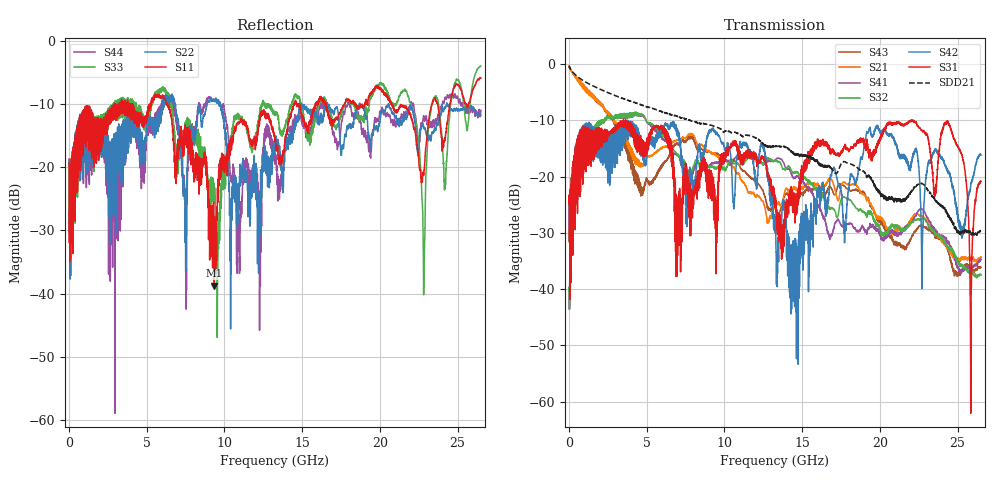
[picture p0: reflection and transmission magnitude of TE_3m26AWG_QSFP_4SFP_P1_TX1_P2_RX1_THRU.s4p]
!Agilent Technologies,N5222A,MY51421691,A.10.00.00
!Agilent N5222A: A.10.00.00
!Date: Friday, January 30, 2015 12:33:07
!Correction: S11(Full 4 Port(1,2,3,4))
!S12(Full 4 Port(1,2,3,4))
!S13(Full 4 Port(1,2,3,4))
!S14(Full 4 Port(1,2,3,4))
!S21(Full 4 Port(1,2,3,4))
!S22(Full 4 Port(1,2,3,4))
!S23(Full 4 Port(1,2,3,4))
!S24(Full 4 Port(1,2,3,4))
!S31(Full 4 Port(1,2,3,4))
!S32(Full 4 Port(1,2,3,4))
!S33(Full 4 Port(1,2,3,4))
!S34(Full 4 Port(1,2,3,4))
!S41(Full 4 Port(1,2,3,4))
!S42(Full 4 Port(1,2,3,4))
!S43(Full 4 Port(1,2,3,4))
!S44(Full 4 Port(1,2,3,4))
!S4P File: Measurements: <S11,S12,S13,S14>,
!<S21,S22,S23,S24>,
!<S31,S32,S33,S34>,
!<S41,S42,S43,S44>:
# Hz S  dB  R 50.0
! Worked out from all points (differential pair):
!   2650 points, 10 MHz to 26.5 GHz, reference 50 ohm
!   strongest paths, dB at 10 MHz, 6.63 GHz, 13.26 GHz, 19.88 GHz, 26.5 GHz:
!     S31: -24.8, -18.2, -24.5, -13.7, -20.9
!     S42: -24.9, -11.0, -27.5, -11.2, -16.2
!     S32: -40.3, -14.9, -17.2, -28.8, -37.5
!     S41: -40.1, -15.6, -17.1, -29.6, -34.7
!     S21: -0.4, -14.0, -25.1, -27.3, -34.3
!     S43: -0.4, -15.2, -25.6, -27.6, -36.1
!   taken as a pair (ports 1,3 in; 2,4 out), SDD21 dB: -0.3, -9.1, -14.6, -22.5, -29.6
!   lowest |S11| = -38.7 dB at 9.35 GHz (marker M1), VSWR 1.02, Z = 51.2 + j0.0243 ohm
!   |S11| at or under -10 dB: start of sweep to 2.939 GHz; 6.306 GHz to 14.46 GHz (8.153 GHz wide, 78.5 % of centre); 20.75 GHz to 23.35 GHz (2.608 GHz wide, 11.8 % of centre)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
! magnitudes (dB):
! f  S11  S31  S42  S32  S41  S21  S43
! 10 MHz  -19.4  -24.8  -24.9  -40.3  -40.1  -0.4  -0.4
! 1.96 GHz  -13.2  -12.0  -11.8  -10.8  -10.9  -6.8  -6.8
! 9.35 GHz  -38.7  -27.7  -11.8  -18.6  -17.6  -15.8  -15.8
! 10.9 GHz  -13.0  -15.3  -16.2  -17.8  -16.4  -19.5  -17.8
! 14.32 GHz  -11.4  -23.8  -43.5  -18.9  -19.6  -22.6  -23.3
! 22.81 GHz  -21.1  -11.8  -26.3  -27.5  -26.0  -27.3  -29.0
! 26.5 GHz  -5.9  -20.9  -16.2  -37.5  -34.7  -34.3  -36.1
